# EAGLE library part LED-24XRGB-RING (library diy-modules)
24 LEDs RGB Ring based on WS2812B More details about controlling WS2812B RGB LEDs are available here: https://learn.sparkfun.com/tutorials/ws2812-breakout-hookup-guide Click here to find device on ebay.com
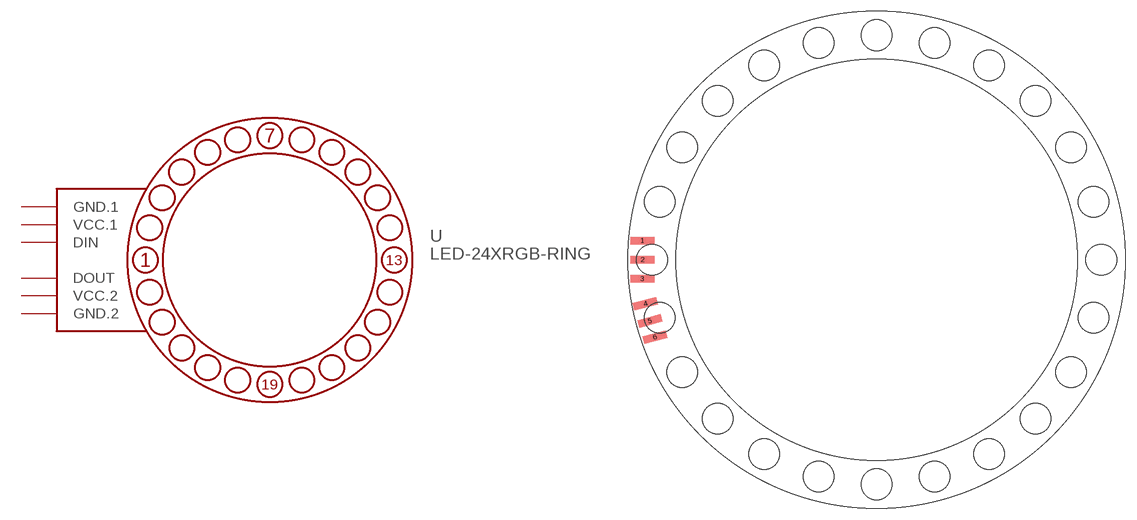
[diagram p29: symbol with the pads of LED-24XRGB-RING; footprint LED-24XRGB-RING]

Designator prefix -

## LED-24XRGB-RING  [LED-24XRGB-RING]
1  GND.1  pwr
2  VCC.1  pwr
3  DIN  in
4  DOUT  in
5  VCC.2  pwr
6  GND.2  pwr

## Footprint LED-24XRGB-RING (pad centres in mm)
24 LEDs RGB Ring based on WS2812B
smd 3.175 x 1.016: 1 -31.115,2.54; 2 -31.115,0; 3 -31.115,-2.54
smd 3.175 x 1.016 rotated 15: 4 -30.734,-5.842; 5 -30.099,-8.128; 6 -29.464,-10.287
